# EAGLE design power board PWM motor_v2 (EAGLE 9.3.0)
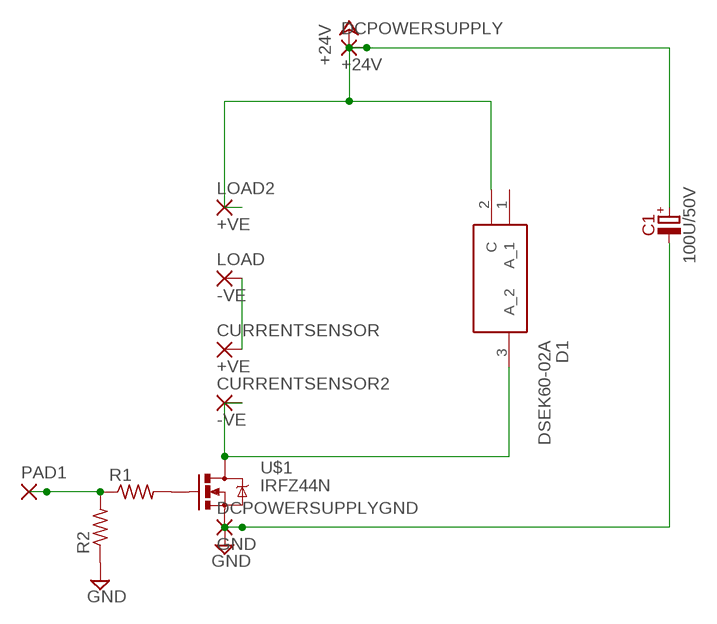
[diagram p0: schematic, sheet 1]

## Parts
C1  100U/50V  [E3,5-8]
CURRENTSENSOR  +VE  SMD5  [SMD2,54-5,08]
CURRENTSENSOR2  -VE  SMD5  [SMD2,54-5,08]
D1  DSEK60-02A  [TO545P530X1600X2596-3P]
DCPOWERSUPPLY  +24V  SMD5  [SMD2,54-5,08]
DCPOWERSUPPLYGND  GND  SMD5  [SMD2,54-5,08]
LOAD  -VE  SMD5  [SMD2,54-5,08]
LOAD2  +VE  SMD5  [SMD2,54-5,08]
PAD1  SMD5  [SMD2,54-5,08]
R1  RES-US1206FAB  [R1206FAB]
R2  RES-US1206FAB  [R1206FAB]
U$1  IRFZ44N  [TO-220]

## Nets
+24V: C1.+ D1.2(C) DCPOWERSUPPLY.1(P) LOAD2.1(P)
GND: C1.- DCPOWERSUPPLYGND.1(P) R2.1 U$1.3(S)
N$1: R1.2 U$1.1(G)
N$2: PAD1.1(P) R1.1 R2.2
N$3: CURRENTSENSOR2.1(P) D1.3(A_2) U$1.2(D)
N$4: CURRENTSENSOR.1(P) LOAD.1(P)
Unconnected: D1.1(A_1)

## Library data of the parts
C1 = capacitors-electrolytic:?; MOUSER: 647-UKA1H101MPD
CURRENTSENSOR CURRENTSENSOR2 DCPOWERSUPPLY DCPOWERSUPPLYGND LOAD LOAD2 PAD1 = wirepad:SMD5: SMD PAD
D1 = SamacSys_Parts:DSEK60-02A: IXYS 200V 50A, Dual Diode, 3-Pin TO-247AD DSEK60-02A Source: Datasheet; DESCRIPTION: IXYS 200V 50A, Dual Diode, 3-Pin TO-247AD DSEK60-02A; HEIGHT: 5.3mm; MANUFACTURER_NAME: IXYS SEMICONDUCTOR; MANUFACTURER_PART_NUMBER: DSEK60-02A; MOUSER_PART_NUMBER: 747-DSEK60-02A; MOUSER_PRICE-STOCK: https://www.mouser.com/Search/Refine.aspx?Keyword=747-DSEK60-02A; RS_PART_NUMBER: 7115326P; RS_PRICE-STOCK: http://uk.rs-online.com/web/p/products/7115326P
R1 R2 = fab:RES-US: Resistor (US Symbol)
U$1 = IRFZ44N:IRFZ44N; AVAILABILITY: Unavailable; DESCRIPTION: Semiconductors and Actives, mosfet, Transistors, Discretes _diodes, transistors, thyristors ..._; MF: Infineon Technologies; MP: IRFZ44N; PACKAGE: D2PAK NXP Semiconductors; PRICE: None

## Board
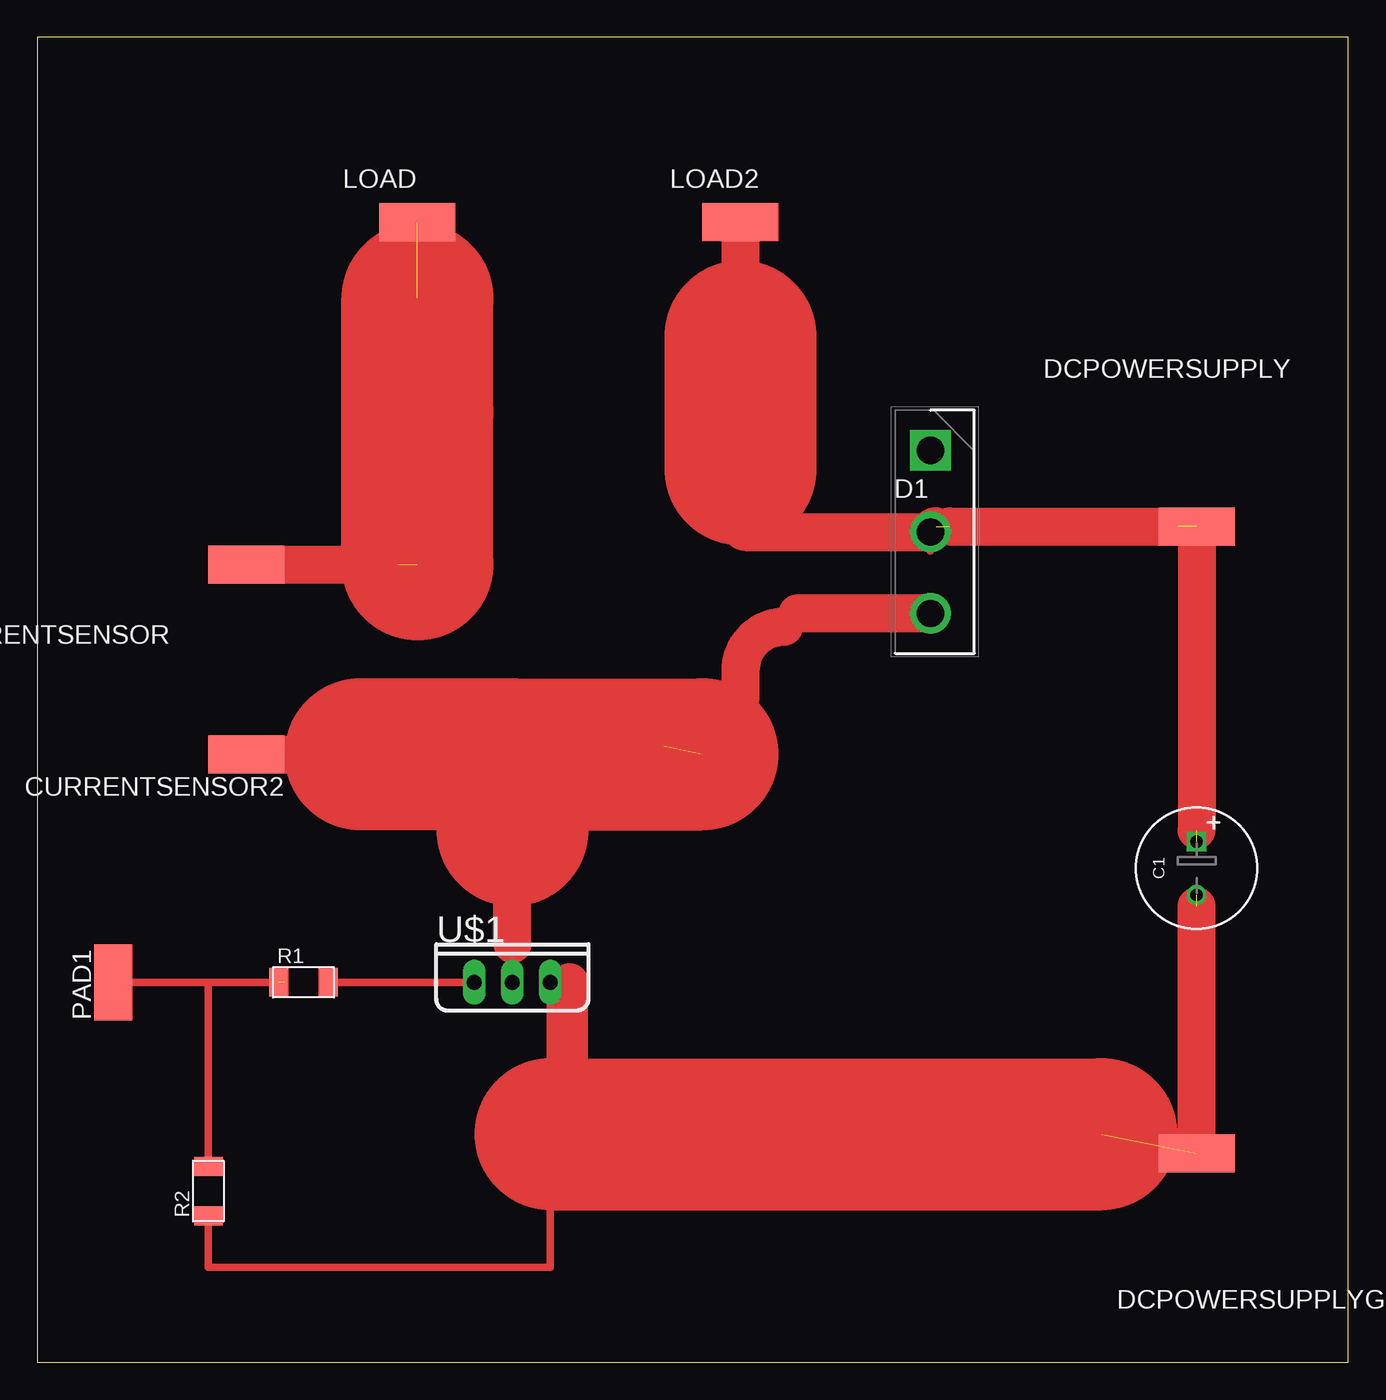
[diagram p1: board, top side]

Size 87.61 x 88.57 mm. Coordinates in mm from the lower left corner, seen from the top.
Outline: 0,0 87.61,0 87.61,88.57 0,88.57 0,0
Copper layers (1*16): Top 0.035mm / dielectric 1.5mm / Bottom 0.035mm
Design rules "default *": minimum track width 20mil, minimum drill 0.35mm, track to track 20mil, track to pad 20mil, pad to pad 20mil, via to via 20mil, smd to smd 20mil, copper to edge 40mil, drill to drill 6mil, minimum pad ring 10mil, minimum via ring 8mil, stop-mask expansion 4mil, vias tented up to drill 0mil, thermal gap 10mil

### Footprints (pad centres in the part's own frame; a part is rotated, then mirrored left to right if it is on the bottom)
E3,5-8 = drill 0.813 square: + -1.778,0 | drill 0.813: - 1.778,0
SMD2,54-5,08 = smd 2.54 x 5.08: 1 0,0
TO545P530X1600X2596-3P = drill 1.81 pad 2.715 square: 1 0,0 | drill 1.81 pad 2.715: 2 5.45,0; 3 10.9,0
R1206FAB = smd 1.27 x 1.905: 1 -1.651,0; 2 1.651,0
TO-220 = drill 1 long: 1 -2.54,0; 2 0,0; 3 2.54,0

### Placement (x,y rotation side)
C1  77.47,33.02 270 top
CURRENTSENSOR  13.97,53.34 90 top
CURRENTSENSOR2  13.97,40.64 90 top
D1  59.69,60.96 270 top
DCPOWERSUPPLY  77.47,55.88 90 top
DCPOWERSUPPLYGND  77.47,13.97 90 top
LOAD  25.4,76.2 90 top
LOAD2  46.99,76.2 90 top
PAD1  5.08,25.4 0 top
R1  17.78,25.4 0 top
R2  11.43,11.43 90 top
U$1  31.75,25.4 0 top

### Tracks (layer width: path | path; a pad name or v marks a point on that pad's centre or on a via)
+24V  (3 unrouted)
  Top 0.508: D1.2 59.69,54.24
  Top 10.16: 46.99,68.58 46.99,59.69
  Top 2.54: 46.99,59.69 46.99,55.88 arc90 47.36,55.51 D1.2 arc-90 60.06,55.88 | LOAD2.1 46.99,68.58 | 60.96,55.88 76.2,55.88 | DCPOWERSUPPLY.1 77.47,35.56
GND  (2 unrouted)
  Top 0.508: R2.1 11.43,6.35 34.29,6.35 34.29,15.24 U$1.3
  Top 10.16: 34.29,15.24 71.12,15.24
  Top 2.54: 34.29,15.24 arc90 35.56,16.51 35.56,25.4 | DCPOWERSUPPLYGND.1 77.47,30.48
N$1
  Top 0.508: R1.2 U$1.1
N$2  (1 unrouted)
  Top 0.508: PAD1.1 11.43,25.4 | 11.43,25.4 16.51,25.4 | R2.2 11.43,25.4
N$3  (1 unrouted)
  Top 0.508: U$1.2 31.75,27.94 | 31.75,35.56 26.67,40.64 24.13,40.64 | 50.8,50.06 49.9,49.16 41.91,41.17 | 26.67,41.17 14.5,41.17 CURRENTSENSOR2.1
  Top 10.16: 31.75,40.64 21.59,40.64 | 31.75,35.56 31.75,40.64 | 31.75,40.64 44.45,40.64
  Top 2.54: 31.75,27.94 31.75,35.56 | D1.3 50.8,50.06 | 49.9,49.16 arc90 46.99,46.25 46.99,44.45 | CURRENTSENSOR2.1 21.59,40.64 24.13,40.64
N$4  (2 unrouted)
  Top 10.16: 25.4,53.34 25.4,63.5 25.4,71.12
  Top 2.54: CURRENTSENSOR.1 24.13,53.34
